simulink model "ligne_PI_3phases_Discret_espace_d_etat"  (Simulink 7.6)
settings: Solver=ode3  StartTime=0.0  StopTime=0.02  RelTol=1e-3
InitFcn:
  | sys = power_analyze('ligne_PI_3phases_Discret','ss');
StopFcn:
  | load Ia_Ua.mat
  | subplot 211
  | plot(x(1,:),x(2,:), x(1,:),x(3,:),x(1,:),x(4,:))
  | grid
  | title('Tensions du système triphasé')
  | xlabel('temps')
  | 
  | subplot 212
  | plot(x(1,:),x(5,:),x(1,:),x(6,:),x(1,:),x(7,:))
  | title('Sorties du modèle d''état')
  | grid
  | xlabel('temps')
libraries: powerlib x11

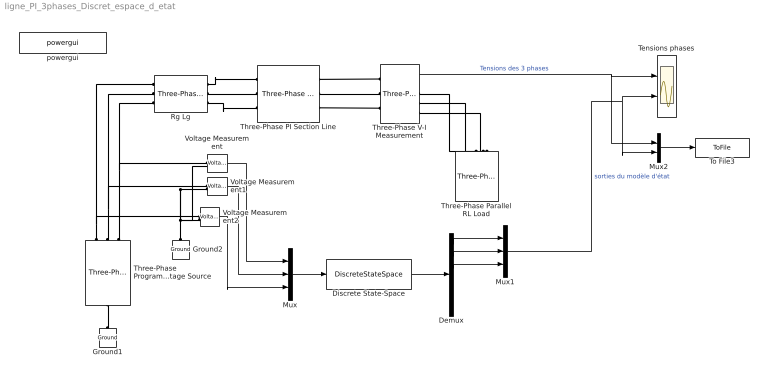
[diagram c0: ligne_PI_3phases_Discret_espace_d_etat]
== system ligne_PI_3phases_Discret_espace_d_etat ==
  Demux : Demux  Outputs=6
  Discrete State-Space : DiscreteStateSpace  A=sys.a  B=sys.b  C=sys.c  D=sys.d  SampleTime=-1
  Ground1 : powerlib/Elements/Ground  DialogController=POWERSYS.PowerSysDialog  PhysicalDomain=powersysdomain  SubClassName=unknown  LeftPortType=p1  RightPortType=p1  LConnTagsString=a
  Ground2 : powerlib/Elements/Ground  DialogController=POWERSYS.PowerSysDialog  PhysicalDomain=powersysdomain  SubClassName=unknown  LeftPortType=p1  RightPortType=p1  LConnTagsString=a
  Mux : Mux  Inputs=3
  Mux1 : Mux  Inputs=3
  Mux2 : Mux  Inputs=2
  Rg Lg : powerlib/Elements/Three-Phase Parallel RLC Branch  DialogController=POWERSYS.PowerSysDialog  PhysicalDomain=powersysdomain  SubClassName=unknown  LeftPortType=p1  RightPortType=p1  LConnTagsString=A|B|C  RConnTagsString=A|B|C  BranchType=RL  Resistance=1  Inductance=1e-3  Capacitance=1e-6  Measurements=None
  Tensions phases : Scope  NumInputPorts=2
  Three-Phase PI Section Line : powerlib/Elements/Three-Phase PI Section Line  DialogController=POWERSYS.PowerSysDialog  PhysicalDomain=powersysdomain  SubClassName=unknown  LeftPortType=p1  RightPortType=p1  LConnTagsString=a|b|c  RConnTagsString=A|B|C  Frequency=60  Resistances=[ 0.01273 0.3864]  Inductances="[ 0.9337e-3  4.1264e-3]"  Capacitances=[12.74e-9 7.751e-9]  Length=150
  Three-Phase Parallel RL Load : powerlib/Elements/Three-Phase Parallel RLC Load  DialogController=POWERSYS.PowerSysDialog  PhysicalDomain=powersysdomain  SubClassName=unknown  LeftPortType=p1  RightPortType=p1  LConnTagsString=A|B|C  Configuration=Y (grounded)  NominalVoltage=230/sqrt(2)  NominalFrequency=60  ActivePower=1e3  InductivePower=10  CapacitivePower=0  Measurements=None
  Three-Phase Programmable Voltage Source : powerlib/Electrical Sources/Three-Phase Programmable Voltage Source  DialogController=POWERSYS.PowerSysDialog  SystemSampleTime=-1  PositiveSequence="[220e6/sqrt(2)  0 60]"  VariationEntity=None  VariationType=Step  VariationStep=0.5  VariationRate=10  VariationMagnitude=0.3  VariationFrequency=2  VariationTiming=[1 2]  VariationPhaseA=off  Amplitudes=[1 0.8 1.2 1.0]  TimeValues=[0 0.1 0.15 0.2]  HarmonicGeneration=off  HarmonicA=[3 0.2 -25 0]  HarmonicB=[2 0.15 35 2]  Timing="[0.05  3]"
  Three-Phase V-I Measurement : powerlib/Measurements/Three-Phase V-I Measurement  DialogController=POWERSYS.PowerSysDialog  SystemSampleTime=-1  VoltageMeasurement=phase-to-ground  SetLabelV=off  LabelV=Vabc  Vpu=off  VpuLL=off  CurrentMeasurement=yes  SetLabelI=off  LabelI=Iabc  Ipu=off  Pbase=100e6  Vbase=500e3  OutputType=Complex  PhasorSimulation=off  PSBequivalent=0
  To File3 : ToFile  Filename=Ia_Ua  MatrixName=x
  Voltage Measurement : powerlib/Measurements/Voltage Measurement  DialogController=POWERSYS.PowerSysDialog  SystemSampleTime=-1  PhasorSimulation=off  OutputType=Complex  PSBequivalent=0
  Voltage Measurement1 : powerlib/Measurements/Voltage Measurement  DialogController=POWERSYS.PowerSysDialog  SystemSampleTime=-1  PhasorSimulation=off  OutputType=Complex  PSBequivalent=0
  Voltage Measurement2 : powerlib/Measurements/Voltage Measurement  DialogController=POWERSYS.PowerSysDialog  SystemSampleTime=-1  PhasorSimulation=off  OutputType=Complex  PSBequivalent=0
  powergui : powerlib/powergui  Priority=1  SystemSampleTime=-1  SimulationMode=Discrete  SampleTime=50e-6  frequency=60  SPID=off  DisableSnubberDevices=off  DisableRonSwitches=off  DisableVfSwitches=off  SwTol=0  Interpol=off  frequencyindice=60  echomessages=off  HookPort=off  DisplayEquations=off  FunctionMessages=off  EnableUseOfTLC=off  x0status=blocks  RestoreLinks=warning  ResistiveCurrentMeasurement=off  Frange=[0:2:200]  Ylog=off  Xlog=on  ShowGrid=on  save=off  variable=ZData  ZoomFFT=off  StartTime=0.0  cycles=1  DisplayStyle=1  fundamental=60  FreqAxis=off  MaxFrequency=1000  frequencyindicesteady=1  display=off  methode=off
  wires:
  Three-Phase V-I Measurement/1 -> Tensions phases/1, Mux2/1  "Tensions des 3 phases"
  Mux/1 -> Discrete State-Space/1
  Voltage Measurement/1 -> Mux/1
  Voltage Measurement1/1 -> Mux/2
  Voltage Measurement2/1 -> Mux/3
  Discrete State-Space/1 -> Demux/1
  Demux/1 -> Mux1/1
  Demux/2 -> Mux1/2
  Demux/3 -> Mux1/3
  Mux1/1 -> Tensions phases/2, Mux2/2  "sorties du modèle d'état"
  Mux2/1 -> To File3/1
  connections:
  Three-Phase Programmable Voltage Source/LConn1 -- Ground1/LConn1
  Three-Phase Programmable Voltage Source/RConn1 -- Rg Lg/LConn1 -- Voltage Measurement2/LConn1
  Three-Phase Programmable Voltage Source/RConn2 -- Rg Lg/LConn2 -- Voltage Measurement1/LConn1
  Three-Phase Programmable Voltage Source/RConn3 -- Rg Lg/LConn3 -- Voltage Measurement/LConn1
  Rg Lg/RConn1 -- Three-Phase PI Section Line/LConn1
  Rg Lg/RConn2 -- Three-Phase PI Section Line/LConn2
  Rg Lg/RConn3 -- Three-Phase PI Section Line/LConn3
  Three-Phase PI Section Line/RConn1 -- Three-Phase V-I Measurement/LConn1
  Three-Phase PI Section Line/RConn2 -- Three-Phase V-I Measurement/LConn2
  Three-Phase PI Section Line/RConn3 -- Three-Phase V-I Measurement/LConn3
  Three-Phase V-I Measurement/RConn3 -- Three-Phase Parallel RL Load/LConn3
  Three-Phase V-I Measurement/RConn2 -- Three-Phase Parallel RL Load/LConn2
  Three-Phase V-I Measurement/RConn1 -- Three-Phase Parallel RL Load/LConn1
  Voltage Measurement/LConn2 -- Voltage Measurement1/LConn2 -- Ground2/LConn1 -- Voltage Measurement2/LConn2
